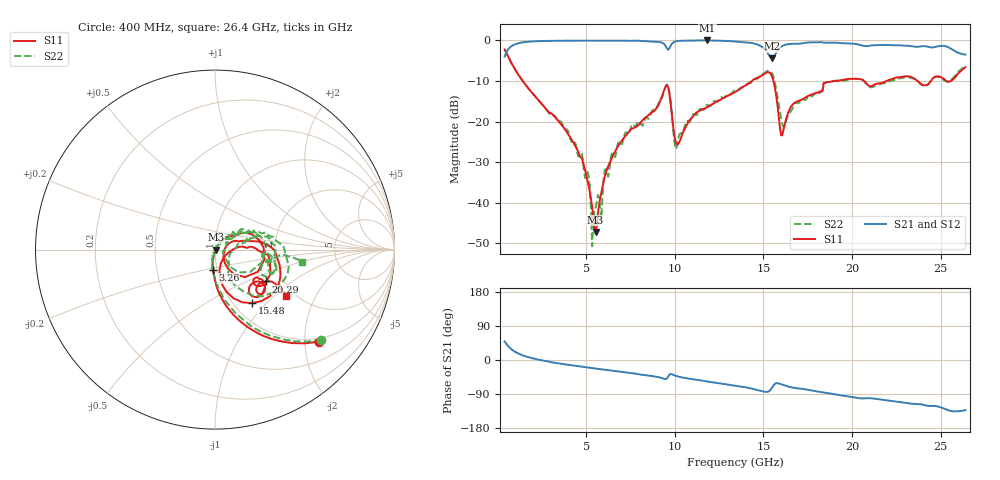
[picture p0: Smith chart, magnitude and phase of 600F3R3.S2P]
!  American Technical Ceramics  Date:  10/23/06
!  One Norden Lane
!  Huntington Station,  NY.  11746-2102
!  Tel:  (631) 622-4700  Fax:  (631) 622-4748
!  Part Number  600F3R3  Mounting Orientation: Horizontal
!  Description: Ultra Low ESR Microwave capacitors
!  Application: Coupling, Bypass, Tuning, DC Block
!  Filters, Matching
# GHZ S DB R 50
! Freq  |S11|  S11 Ph  |S21|  S21 Ph  |S12|  S12 Ph  |S22|  S22 Ph
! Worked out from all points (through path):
!   401 points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, 400 MHz to 26.4 GHz, reference 50 ohm
!   highest |S21| = -0.01 dB at 11.84 GHz (marker M1); lowest = -4.4 dB at 15.48 GHz (marker M2)
!   group delay of S21, straight-line fit = 15.3 ps
!   lowest |S11| = -47.2 dB at 5.535 GHz (marker M3), VSWR 1.01, Z = 50.4 - j0.108 ohm
!   |S11| at or under -10 dB: 1.42 GHz to 14.35 GHz (12.93 GHz wide, 164 % of centre); 15.57 GHz to 19.03 GHz (3.462 GHz wide, 20 % of centre); 20.69 GHz to 21.95 GHz (1.268 GHz wide, 5.95 % of centre)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
!   |S22| runs from -50.7 to -2.2 dB; largest |S21 - S12| = 0.0058
!   S11 on the Smith chart (normalised r, x): 400 MHz: 0.91, -2.33; 3.26 GHz: 0.95, -0.22; 15.48 GHz: 1.21, -0.83; 20.29 GHz: 1.64, -0.66; 26.4 GHz: 1.79, -1.19
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0.4  -2.23 -41.5  -4.00 48.9  -3.99 49.0  -2.21 -40.3
1.245  -8.90 -75.6  -0.62 15.7  -0.61 15.6  -8.86 -72.9
3.26  -18.92 -97.0  -0.10 -7.5  -0.09 -7.6  -18.71 -93.6
4.755  -29.02 -100.8  -0.06 -17.7  -0.05 -17.8  -27.81 -103.5
5.405  -43.43 -69.1  -0.05 -21.7  -0.05 -21.8  -44.21 -143.9
5.535  -47.22 -14.3  -0.05 -22.5  -0.05 -22.7  -41.46 -55.0
6.12  -32.51 54.5  -0.05 -26.0  -0.04 -26.1  -31.75 62.6
6.64  -27.33 56.4  -0.05 -29.2  -0.05 -29.4  -28.77 55.5
9.11  -15.71 33.0  -0.39 -45.5  -0.40 -45.6  -15.11 37.8
9.63  -11.42 -27.5  -2.32 -43.8  -2.33 -44.0  -11.37 -15.2
10.085  -25.43 -24.8  -0.21 -42.2  -0.21 -42.3  -26.73 -10.5
11.84  -16.45 18.4  -0.01 -56.7  -0.01 -56.7  -15.84 35.0
13.4  -12.73 11.4  -0.26 -67.8  -0.27 -67.9  -12.29 26.2
14.7  -9.16 -7.4  -1.08 -79.6  -1.08 -79.6  -9.29 8.6
15.48  -8.80 -55.2  -4.41 -73.6  -4.42 -73.6  -8.04 -37.5
16.065  -23.40 -26.1  -1.37 -65.1  -1.38 -65.1  -20.60 -33.1
16.65  -15.83 5.1  -0.83 -72.7  -0.83 -72.7  -16.77 13.0
17.755  -13.30 2.6  -0.48 -80.9  -0.48 -80.9  -13.80 18.8
20.29  -9.47 -31.9  -0.93 -100.0  -0.94 -100.0  -9.50 -1.8
22.11  -9.70 -33.9  -1.17 -107.4  -1.17 -107.3  -10.10 -5.9
25.425  -10.14 -41.2  -1.65 -132.4  -1.64 -132.6  -10.25 -15.4
26.4  -6.56 -33.3  -3.48 -132.3  -3.51 -132.2  -6.24 -8.3
